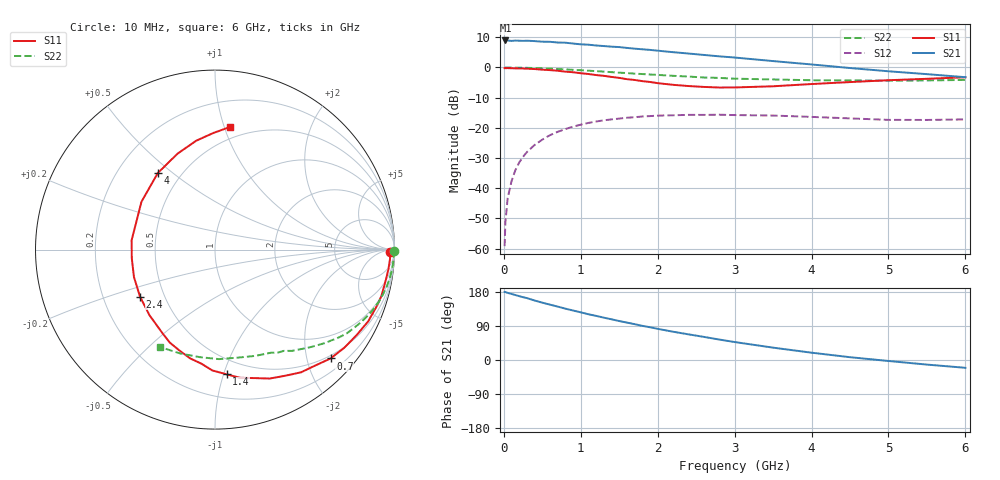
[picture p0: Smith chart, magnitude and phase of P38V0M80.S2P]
! SIEMENS Small Signal Semiconductors
! BFP181
! Si NPN RF Bipolar Junction Transistor in SOT143
! VCE = 8 V  IC = 0.8 mA
! Common Emitter S-Parameters:  March  1996
# GHz  S  MA  R  50
!  f  S11  S21  S12  S22
! GHz  MAG  ANG  MAG  ANG  MAG  ANG  MAG  ANG
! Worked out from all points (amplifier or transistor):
!   36 points, 10 MHz to 6 GHz, reference 50 ohm
!   highest |S21| = 9.0 dB at 20 MHz (marker M1)
!   |S21| within 3 dB of that: start of sweep to 1.839 GHz
!   unconditionally stable (mu >= 1): 3.487 GHz to end of sweep
!   at 250 MHz: K = 0.09, MSG = 19.2 dB, |S12| = -29.6 dB
!   at 1.4 GHz: K = 0.45, MSG = 12.0 dB, |S12| = -17.2 dB
!   at 6 GHz: K = 1.31, MAG = 3.6 dB, |S12| = -17.2 dB
!   S11 on the Smith chart (normalised r, x): 10 MHz: 62, -35; 700 MHz: 0.44, -2.45; 1.4 GHz: 0.38, -1.02; 2.4 GHz: 0.36, -0.25; 4 GHz: 0.37, +0.44; 6 GHz: 0.40, +1.05
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0.01  0.9759 -0.8  2.778 179.5  0.0011 84.2  0.9991 -0.3
0.02  0.9747 -1.4  2.804 179.4  0.0027 87.7  0.9969 -0.6
0.05  0.9766 -3.0  2.798 177.1  0.0069 89.3  0.9967 -1.5
0.1  0.9726 -6.4  2.757 174.4  0.0131 85.9  0.9959 -3.0
0.2  0.9637 -12.5  2.775 168.5  0.0268 81.0  0.9928 -6.0
0.3  0.9556 -19.0  2.779 163.4  0.0398 76.8  0.9871 -9.1
0.4  0.9425 -25.1  2.736 157.0  0.0522 72.8  0.9794 -12.0
0.6  0.9041 -37.3  2.664 146.1  0.0758 64.7  0.9585 -17.6
0.7  0.8845 -43.3  2.593 140.9  0.0861 60.6  0.9438 -20.4
0.8  0.8532 -49.3  2.575 135.5  0.0956 56.8  0.9307 -22.8
1.1  0.7804 -67.0  2.386 120.7  0.1209 46.3  0.8852 -29.9
1.4  0.6978 -84.7  2.213 107.4  0.1384 36.8  0.8374 -36.4
1.5  0.6733 -91.3  2.179 102.8  0.1427 34.2  0.8209 -38.1
1.8  0.5947 -109.8  2.003 90.1  0.1544 26.9  0.7792 -43.2
2.2  0.5166 -135.0  1.793 74.6  0.1617 18.0  0.7281 -49.8
2.4  0.4932 -147.9  1.704 67.7  0.1644 13.9  0.7084 -52.8
3  0.4674 173.6  1.463 47.4  0.163 4.7  0.6533 -61.6
3.5  0.4887 147.0  1.277 32.6  0.1601 -1.1  0.6336 -69.1
4  0.5324 126.8  1.123 19.3  0.152 -5.0  0.6153 -77.9
4.5  0.5736 111.4  0.98 7.4  0.1437 -8.0  0.6106 -87.9
5.5  0.6498 90.8  0.776 -12.1  0.1354 -4.6  0.6104 -108.5
6  0.6889 82.9  0.691 -20.6  0.1383 -3.1  0.6227 -119.3
